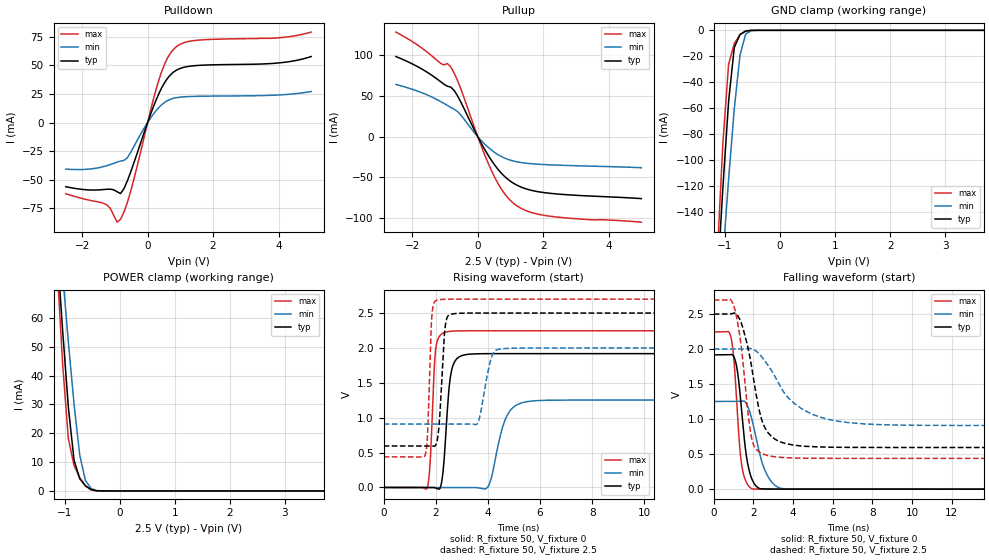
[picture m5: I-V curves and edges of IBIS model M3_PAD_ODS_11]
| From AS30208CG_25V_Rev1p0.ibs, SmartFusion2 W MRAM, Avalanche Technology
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[Model] M3_PAD_ODS_11
Model_type I/O
Enable   Active-High
Vinl  =  0.7
Vinh  =  1.8
Vmeas =  1.25
Cref  =  30e-12
| Capacitance   typ   min   max
C_comp   1.569373e-12  1.477665e-12  1.713725e-12
| Variables   typ   min   max
[GND Clamp Reference]   0   0   0
[POWER Clamp Reference]   2.5   2   2.7
[Pulldown Reference]   0   0   0
[Pullup Reference]   2.5   2   2.7
[Temperature Range]   25   125   -40
[Voltage Range]   2.5   2   2.7
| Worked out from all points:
|   slope of the pulldown table from 0 to 0.375 V, typ, clamps not added: 13.9 ohm
|   slope of the pullup table from 0 to 0.375 V, typ, clamps not added: 14.2 ohm
|   GND clamp passes 1 mA (typ) near -0.64 V on its own axis
|   POWER clamp passes 1 mA (typ) near -0.56 V on its own axis
|   falling waveform, R_fixture 50, V_fixture 0: 20-80 % time 435ps typ, 692ps min, 330ps max; typ from 1.92 V to 0 V
|   falling waveform, R_fixture 50, V_fixture 2.5: 20-80 % time 793ps typ, 1.86ns min, 531ps max; typ from 2.5 V to 0.595 V
|   rising waveform, R_fixture 50, V_fixture 0: 20-80 % time 227ps typ, 494ps min, 157ps max; typ from 0 V to 1.92 V
|   rising waveform, R_fixture 50, V_fixture 2.5: 20-80 % time 174ps typ, 325ps min, 121ps max; typ from 0.595 V to 2.5 V
[GND Clamp]
| Voltage   I(typ)   I(min)   I(max)
-2.5V     -1.297A    -1.146A    -1.538A
-1.138V   -196mA     -238.3mA   -175.4mA
-1.034V   -121.2mA   -175.1mA   -86.76mA
-931mV    -54.83mA   -114.9mA   -26.21mA
-827.6mV  -13.18mA   -60.42mA   -10.12mA
-724.1mV  -3.226mA   -19.15mA   -3.372mA
-620.7mV  -623.1uA   -2.801mA   -433.9uA
-517.2mV  -35.15uA   -320.3uA   -7.309uA
-413.8mV  -841.1nA   -24.53uA   -57.63nA
5V        0A         0A         0A
[POWER Clamp]
| Voltage   I(typ)   I(min)   I(max)
-2.5V     511mA      454.9mA    606.6mA
-1.138V   84.76mA    99.9mA     78.64mA
-1.034V   55.67mA    75.27mA    43.94mA
-931mV    29.07mA    51.7mA     18.16mA
-827.6mV  10.68mA    30.08mA    8.788mA
-724.1mV  4.238mA    12.45mA    4.618mA
-620.7mV  1.771mA    3.587mA    1.776mA
-517.2mV  465uA      837.9uA    329.7uA
-413.8mV  47.65uA    120.2uA    11.19uA
-310.3mV  1.515uA    11.72uA    116.8nA
5V        0A         0A         0A
[Pulldown]
| Voltage   I(typ)   I(min)   I(max)
-2.5V     -55.99mA   -40.65mA   -62.12mA
-1.345V   -58.47mA   -38.45mA   -70.46mA
-1.138V   -58.16mA   -36.63mA   -75.08mA
-931mV    -60.43mA   -34.49mA   -86.96mA
-827.6mV  -61.95mA   -33.61mA   -84.4mA
-517.2mV  -43.17mA   -26.04mA   -59.93mA
344.8mV   25.28mA    13.14mA    37.23mA
603.4mV   38.43mA    19.08mA    56.07mA
948.3mV   46.68mA    21.99mA    67.55mA
1.638V    49.99mA    22.96mA    72.11mA
3.99V     51.98mA    24.03mA    73.9mA
5V        57.62mA    27.08mA    78.94mA
[Pullup]
| Voltage   I(typ)   I(min)   I(max)
-2.5V     98.48mA    64.18mA    128.6mA
-1.759V   84.36mA    54.81mA    110.5mA
-1.138V   67.71mA    43.27mA    90.34mA
-827.6mV  61.02mA    35.96mA    86.03mA
-517.2mV  42.65mA    26.62mA    58.92mA
86.21mV   -6.586mA   -3.865mA   -9.317mA
431mV     -29.95mA   -16.92mA   -42.83mA
775.9mV   -47.25mA   -25.57mA   -67.74mA
1.121V    -58.06mA   -30.33mA   -82.9mA
1.552V    -65.2mA    -33.03mA   -92.22mA
2.155V    -69.51mA   -34.62mA   -97.61mA
5V        -76.28mA   -38.29mA   -105.3mA
[Ramp]
dV/dt_r   1.1507/0.226868n  0.751452/0.493824n  1.3472/0.15678n
dV/dt_f   1.14297/0.792955n  0.654868/1.86417n  1.35646/0.531393n
R_load = 50
[Falling Waveform]
R_fixture = 50
V_fixture = 0
V_fixture_min = 0
V_fixture_max = 0
| Time   V(typ)   V(min)   V(max)
0s        1.918V     1.252V     2.245V
863.1ps   1.922V     1.253V     2.173V
1.008ns   1.893V     1.253V     1.872V
1.149ns   1.759V     1.253V     1.288V
1.396ns   1.145V     1.256V     366.3mV
1.625ns   511.9mV    1.231V     107.8mV
1.907ns   155.3mV    1.013V     7.544mV
2.59ns    2.265mV    262.4mV    900uV
3.378ns   775.9uV    12.89mV    863.2uV
21.88ns   -493.9nV   84.59nV    510.3nV
[Falling Waveform]
R_fixture = 50
V_fixture = 2.5
V_fixture_min = 2
V_fixture_max = 2.7
| Time   V(typ)   V(min)   V(max)
0s        2.5V       2V         2.7V
1.029ns   2.513V     2.001V     2.601V
1.374ns   2.382V     2.001V     2.066V
1.883ns   1.789V     2.007V     762.6mV
2.25ns    1.182V     1.944V     540.4mV
2.496ns   928mV      1.861V     500.3mV
3.027ns   725.2mV    1.638V     464.1mV
4.001ns   630.3mV    1.238V     445.1mV
6.284ns   597.7mV    969.1mV    440.1mV
21.88ns   595.1mV    908.6mV    439.2mV
[Rising Waveform]
R_fixture = 50
V_fixture = 0
V_fixture_min = 0
V_fixture_max = 0
| Time   V(typ)   V(min)   V(max)
0s        1.99nV     39.47nV    1.611nV
1.665ns   872.2uV    -346uV     -11.65mV
1.995ns   -8.629mV   -414.8uV   1.978V
2.216ns   57.39mV    -460.6uV   2.197V
2.4ns     855.1mV    -498.9uV   2.229V
2.813ns   1.847V     -584.7uV   2.243V
3.989ns   1.917V     2.846mV    2.245V
4.695ns   1.918V     999.7mV    2.245V
5.487ns   1.918V     1.229V     2.245V
21.88ns   1.918V     1.252V     2.245V
[Rising Waveform]
R_fixture = 50
V_fixture = 2.5
V_fixture_min = 2
V_fixture_max = 2.7
| Time   V(typ)   V(min)   V(max)
0s        595.1mV    908.6mV    439.2mV
1.596ns   594.8mV    909mV      470.8mV
1.685ns   594.8mV    909mV      771.4mV
1.855ns   594.8mV    909.1mV    2.477V
2.068ns   701.7mV    909.1mV    2.686V
2.36ns    2.3V       909.2mV    2.697V
2.609ns   2.484V     909.3mV    2.699V
3.594ns   2.499V     915.7mV    2.699V
4.452ns   2.499V     1.983V     2.699V
21.88ns   2.5V       2V         2.7V
